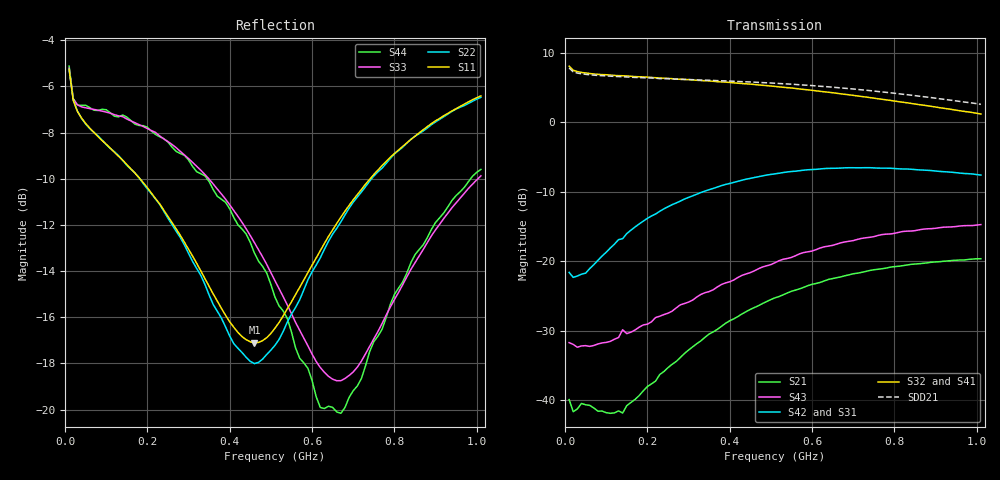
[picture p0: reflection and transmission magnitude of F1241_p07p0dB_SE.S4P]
! Integrated Device Technology
! Corporate Headquarters
! 6024 Silver Creek Valley Road
! San Jose, CA 95138  USA
! Phone:  1-408-284-8200
! Toll Free:  1-800-223-1366
! Webpage:  http://www.idt.com/
! Timing and RF Division
! 515 Groton Road, Suite 102
! Westford, MA 01886-6024
! Device:  F1241
! Description: Dual Intermediate Frequency Digital Variable Gain Amplifier
! Frequency:  10.0 -  500.00 MHz
! Package:  5x5 mm QFN Plastic Package: 32 pin
! Ports:  8 RF, 20 DC
!  Pin  1  = GA3  Pin 17  = RF OUT_B+
!  Pin  2  = GA4  Pin 18  = RF OUT_B-
!  Pin  3  = GA5  Pin 19  = STBY_B
!  Pin  4  = ISET_A  Pin 20  = Ground
!  Pin  5  = ISET_B  Pin 21  = Ground
!  Pin  6  = GB5  Pin 22  = STB_A
!  Pin  7  = GB4  Pin 23  = RF OUT_A-  = Port 4
!  Pin  8  = GB3  Pin 24  = RF OUT_A+  = Port 3
!  Pin  9  = GB2  Pin 25  = NO CONNECT
!  Pin 10  = GB1  Pin 26  = NO CONNECT
!  Pin 11  = RF IN_B+  Pin 27  = VCC
!  Pin 12  = RF IN_B-  Pin 28  = Ground
!  Pin 13  = Ground  Pin 29  = RF IN_A-  = Port 2
!  Pin 14  = VCC  Pin 30  = RF IN_A+  = Port 1
!  Pin 15  = NO CONNECT  Pin 31  = GA1
!  Pin 16  = NO CONNECT  Pin 32  = GA2
! State:  13
! Gain State:  7.0 dB
! Voltages:  Vcc = +5.00 Volts  Icc approximately 160.0 mA or 80 mA per channel.
! Data:  The device was measured on a custom evaluation board which has
!  individual transmission lines to the RF pins.  Data was collected
!  using a calibrated network analyzer.  The evaluation board was
!  de-embedded using a port reference technique.
!  The reference plane is the edge of the package pin.
!  Only Channel A was measured.
!  This data is in single-ended operation.  If your needs are balanced
!  or differential S-parameters then this file needs to be used a
!  linear simulator.
! Misc:  Lot Code  160028MY
!  Action Tracker AT004
! Date Measured:  2014-08-14
! Date:  2014-08-28  MJV
! Note:
!  Integrated Device Technology supplies this data as a sample of measured
!  data at the package pin for this product.  Your particular data for this
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# Hz S dB R 50
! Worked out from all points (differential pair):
!   101 points, 10 MHz to 1.01 GHz, reference 50 ohm
!   strongest paths, dB at 10 MHz, 260 MHz, 510 MHz, 760 MHz, 1.01 GHz:
!     S32: 8.0, 6.2, 5.1, 3.4, 1.2
!     S41: 8.1, 6.2, 5.1, 3.2, 1.0
!     S42: -21.6, -11.9, -7.5, -6.6, -7.6
!     S31: -21.6, -11.8, -7.4, -6.7, -7.7
!     S43: -31.7, -27.2, -20.2, -16.3, -14.8
!     S21: -39.9, -34.9, -25.3, -21.2, -19.7
!   taken as a pair (ports 2,1 in; 3,4 out), SDD21 dB: 7.8, 6.2, 5.6, 4.4, 2.5
!   lowest |S11| = -17.1 dB at 460 MHz (marker M1), VSWR 1.32, Z = 40.5 - j8.37 ohm
!   |S11| at or under -10 dB: 182.1 MHz to 741.1 MHz (558.9 MHz wide, 121 % of centre)
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1e7  -5.25 -23.7  -39.87 -32.5  -69.23 137.4  -16.76 16.0
     -39.94 -31.1  -5.27 -23.4  -16.79 15.6  -70.22 130.7
     -21.60 158.1  8.04 176.5  -5.21 -22.5  -31.91 -174.9
     8.07 176.6  -21.64 158.3  -31.74 -175.3  -5.12 -22.6
2e7  -6.60 -19.4  -41.73 -8.5  -54.76 104.8  -16.54 6.1
     -41.68 -8.3  -6.58 -19.0  -16.60 6.1  -55.39 103.6
     -22.30 145.7  7.46 174.0  -6.53 -14.8  -32.16 176.5
     7.50 173.9  -22.35 145.9  -32.00 176.3  -6.53 -15.0
3e7  -7.07 -18.4  -41.35 3.9  -51.04 94.8  -16.59 2.0
     -41.28 3.2  -7.07 -18.0  -16.61 2.3  -51.26 94.4
     -22.13 135.3  7.26 172.5  -6.79 -11.5  -32.55 172.1
     7.30 172.3  -22.16 135.6  -32.40 172.4  -6.80 -11.2
9e7  -8.34 -24.9  -41.43 22.6  -41.58 78.8  -16.90 -5.4
     -41.58 20.2  -8.32 -24.0  -16.85 -5.1  -41.60 79.6
     -19.22 97.5  6.83 164.1  -7.07 -12.1  -32.12 159.6
     6.84 163.7  -19.28 97.5  -31.78 158.2  -6.99 -11.2
4.6e8  -17.10 -133.4  -26.28 73.4  -28.87 40.2  -16.35 -28.0
       -26.69 76.1  -18.01 -132.6  -16.25 -27.9  -28.86 37.9
       -7.97 17.7  5.40 113.1  -12.76 -57.7  -21.91 106.4
       5.34 112.4  -7.98 16.8  -21.41 105.6  -13.21 -55.9
6.7e8  -11.66 150.1  -22.11 53.1  -26.44 21.8  -16.36 -45.6
       -22.28 56.8  -11.87 148.0  -16.12 -45.7  -26.47 18.0
       -6.64 -17.8  4.06 85.9  -18.74 -136.0  -17.98 77.6
       3.96 85.1  -6.62 -19.5  -17.37 76.3  -20.16 -143.0
1.01e9  -6.41 114.3  -19.89 24.9  -24.30 -7.1  -17.68 -72.2
        -19.67 27.1  -6.47 113.4  -17.21 -72.8  -24.40 -11.8
        -7.71 -61.9  1.16 48.5  -9.87 140.1  -15.27 36.1
        0.99 47.9  -7.63 -65.0  -14.75 35.1  -9.59 135.5
